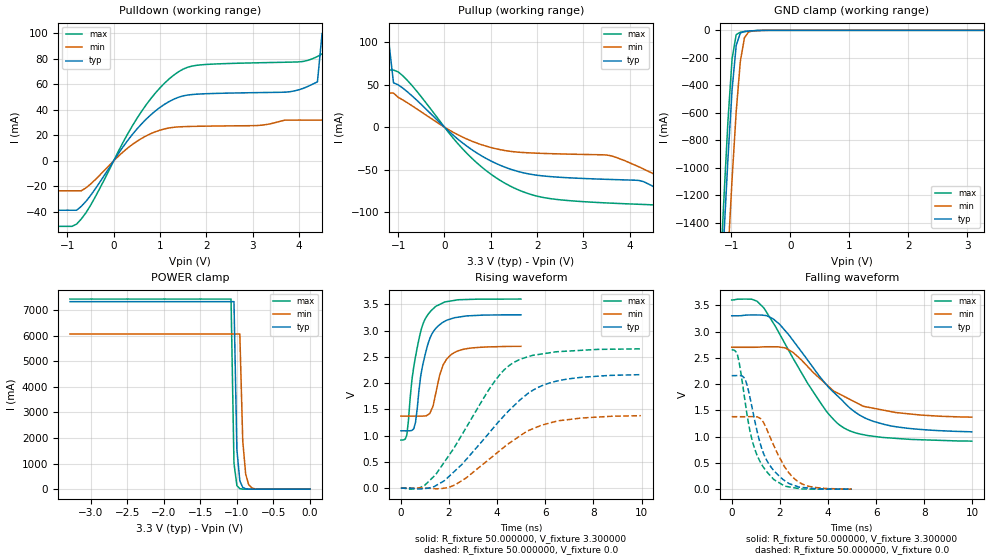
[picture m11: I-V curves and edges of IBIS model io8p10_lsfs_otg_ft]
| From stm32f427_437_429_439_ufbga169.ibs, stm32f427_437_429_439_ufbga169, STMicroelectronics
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|   Model io8p10_lsfs_otg_ft
[Model]  io8p10_lsfs_otg_ft
Model_type I/O
Polarity   Non-Inverting
Enable   Active-Low
Vinl =   0.990000V
Vinh =   2.310000V
Vmeas =  1.650000V
Cref =   40.000000pF
Rref =   100.000000M
Vref =   0.0V
C_comp   8.196500pF   7.968500pF   8.492600pF
[Temperature Range]   25.000000   0.125000k   -40.000000
[Pullup Reference]   3.300000V   2.700000V   3.600000V
[Pulldown Reference]   0.0V   0.0V   0.0V
[POWER Clamp Reference]   3.300000V   2.700000V   3.600000V
[GND Clamp Reference]   0.0V   0.0V   0.0V
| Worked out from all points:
|   slope of the pulldown table from 0 to 0.495 V, typ, clamps not added: 20.1 ohm
|   slope of the pullup table from 0 to 0.495 V, typ, clamps not added: 21.8 ohm
|   GND clamp passes 1 mA (typ) near -0.52 V on its own axis
|   POWER clamp passes 1 mA (typ) near -0.81 V on its own axis
|   rising waveform, R_fixture 50.000000, V_fixture 3.300000: 20-80 % time 528ps typ, 500ps min, 531ps max; typ from 1.09 V to 3.3 V
|   rising waveform, R_fixture 50.000000, V_fixture 0.0: 20-80 % time 2.59ns typ, 2.41ns min, 2.19ns max; typ from 0 V to 2.16 V
|   falling waveform, R_fixture 50.000000, V_fixture 3.300000: 20-80 % time 2.44ns typ, 2.26ns min, 2.13ns max; typ from 3.3 V to 1.09 V
|   falling waveform, R_fixture 50.000000, V_fixture 0.0: 20-80 % time 849ps typ, 951ps min, 758ps max; typ from 2.16 V to 0 V
[Pulldown]
|Voltage   I(typ)   I(min)   I(max)
-3.3V     -38.65mA   -23.43mA   -51.3mA
-800mV    -38.65mA   -23.43mA   -49.55mA
600mV     28.89mA    17.56mA    38.66mA
1.4V      49.88mA    26.66mA    69.85mA
4.1V      56.96mA    32mA       77.99mA
4.4V      62mA       32mA       81.81mA
4.5V      100mA      32mA       83.91mA
4.7V      100mA      32mA       89mA
4.8V      100mA      32mA       100mA
5.1V      100mA      32mA       100mA
5.2V      1A         1A         100mA
6.6V      1A         1A         1A
[Pullup]
|Voltage   I(typ)   I(min)   I(max)
-3.3V     100mA      1A         67mA
-1.6V     100mA      1A         67mA
-1.5V     100mA      40mA       67mA
-1.2V     100mA      40mA       67mA
-1.1V     52mA       40mA       67mA
800mV     -33.66mA   -20.62mA   -46.63mA
2V        -56.45mA   -30.57mA   -80.98mA
3.5V      -61.24mA   -32.7mA    -88.93mA
4.2V      -62.54mA   -46.6mA    -90.53mA
4.9V      -81.9mA    -66mA      -102.4mA
5.5V      -103mA     -66mA      -126.3mA
6.6V      -103mA     -66mA      -139mA
[GND_clamp]
|Voltage   I(typ)   I(min)   I(max)
-3.3V     -9.479A    -9.465A    -9.974A
-1.2V     -2.125A    -2.854A    -1.857A
-1.13V    -1.511A    -2.236A    -1.236A
-1.06V    -933.3mA   -1.641A    -660.9mA
-990mV    -433.3mA   -1.082A    -206.9mA
-920mV    -110.3mA   -591mA     -31.45mA
-850mV    -19.78mA   -226.7mA   -13.65mA
-780mV    -8.311mA   -53.93mA   -9.506mA
-710mV    -5.285mA   -11.94mA   -6.262mA
-640mV    -3.232mA   -4.282mA   -3.577mA
3.28V     0A         0A         0A
[POWER_clamp]
|Voltage   I(typ)   I(min)   I(max)
-3.28V    7.328A     6.064A     7.43A
-1.08V    7.328A     6.064A     7.43A
-1.04V    7.328A     6.064A     1.015A
-1V       1.545A     6.064A     138.6mA
-960mV    325.6mA    6.064A     18.93mA
-920mV    68.64mA    1.89A      2.585mA
-880mV    14.47mA    589mA      353uA
-840mV    3.05mA     183.6mA    105.2uA
-800mV    642.9uA    57.21mA    105.2uA
-720mV    28.59uA    5.557mA    105.2uA
0V        0A         0A         0A
[Ramp]
| variable   typ   min   max
dV/dt_r  1.28459/2.58468n   0.82104/2.39008n   1.58779/2.18681n
dV/dt_f  1.30068/2.41606n   0.78276/2.24376n   1.59783/2.12438n
R_load = 50.000000
[Rising Waveform]
R_fixture= 50.000000
V_fixture= 3.300000
V_fixture_min= 2.700000
V_fixture_max= 3.600000
|time   V(typ)   V(min)   V(max)
0s        1.091V     1.371V     914.6mV
250.2ps   1.091V     1.371V     1.024V
460.5ps   1.099V     1.371V     2.068V
540.5ps   1.139V     1.371V     2.319V
610.6ps   1.261V     1.37V      2.507V
900.9ps   2.328V     1.371V     3.101V
1.251ns   2.899V     1.472V     3.377V
1.752ns   3.159V     2.341V     3.529V
2.142ns   3.232V     2.558V     3.568V
4.985ns   3.3V       2.7V       3.6V
[Rising Waveform]
R_fixture= 50.000000
V_fixture= 0.0
V_fixture_min= 0.0
V_fixture_max= 0.0
|time   V(typ)   V(min)   V(max)
0s        34.9uV     19.6uV     -14.07uV
760.8ps   -17.13mV   32.37uV    1.992mV
1.441ns   43.89mV    -12.78mV   253.8mV
2.242ns   325.6mV    58.21mV    790.1mV
3.704ns   1.071V     563.1mV    1.909V
4.224ns   1.346V     756.5mV    2.22V
4.705ns   1.572V     918.3mV    2.397V
5.526ns   1.875V     1.138V     2.532V
6.466ns   2.037V     1.274V     2.597V
9.97ns    2.161V     1.379V     2.652V
[Falling Waveform]
R_fixture= 50.000000
V_fixture= 3.300000
V_fixture_min= 2.700000
V_fixture_max= 3.600000
|time   V(typ)   V(min)   V(max)
0s        3.3V       2.7V       3.6V
1.041ns   3.315V     2.701V     3.579V
1.722ns   3.241V     2.71V      3.166V
2.543ns   2.833V     2.604V     2.496V
3.644ns   2.149V     2.114V     1.675V
4.104ns   1.902V     1.922V     1.39V
4.645ns   1.663V     1.771V     1.17V
5.325ns   1.406V     1.61V      1.05V
6.346ns   1.231V     1.5V       981.7mV
9.97ns    1.091V     1.371V     914.6mV
[Falling Waveform]
R_fixture= 50.000000
V_fixture= 0.0
V_fixture_min= 0.0
V_fixture_max= 0.0
|time   V(typ)   V(min)   V(max)
0s        2.161V     1.379V     2.652V
250.2ps   2.163V     1.379V     2.536V
580.6ps   2.063V     1.379V     1.594V
750.8ps   1.765V     1.38V      1.122V
961ps     1.298V     1.38V      758.8mV
1.231ns   796.2mV    1.325V     480.6mV
1.522ns   496.6mV    1.069V     296.6mV
2.192ns   164.8mV    428.9mV    60.43mV
2.763ns   44.36mV    141.3mV    12.78mV
4.985ns   34.9uV     19.6uV     -14.07uV
